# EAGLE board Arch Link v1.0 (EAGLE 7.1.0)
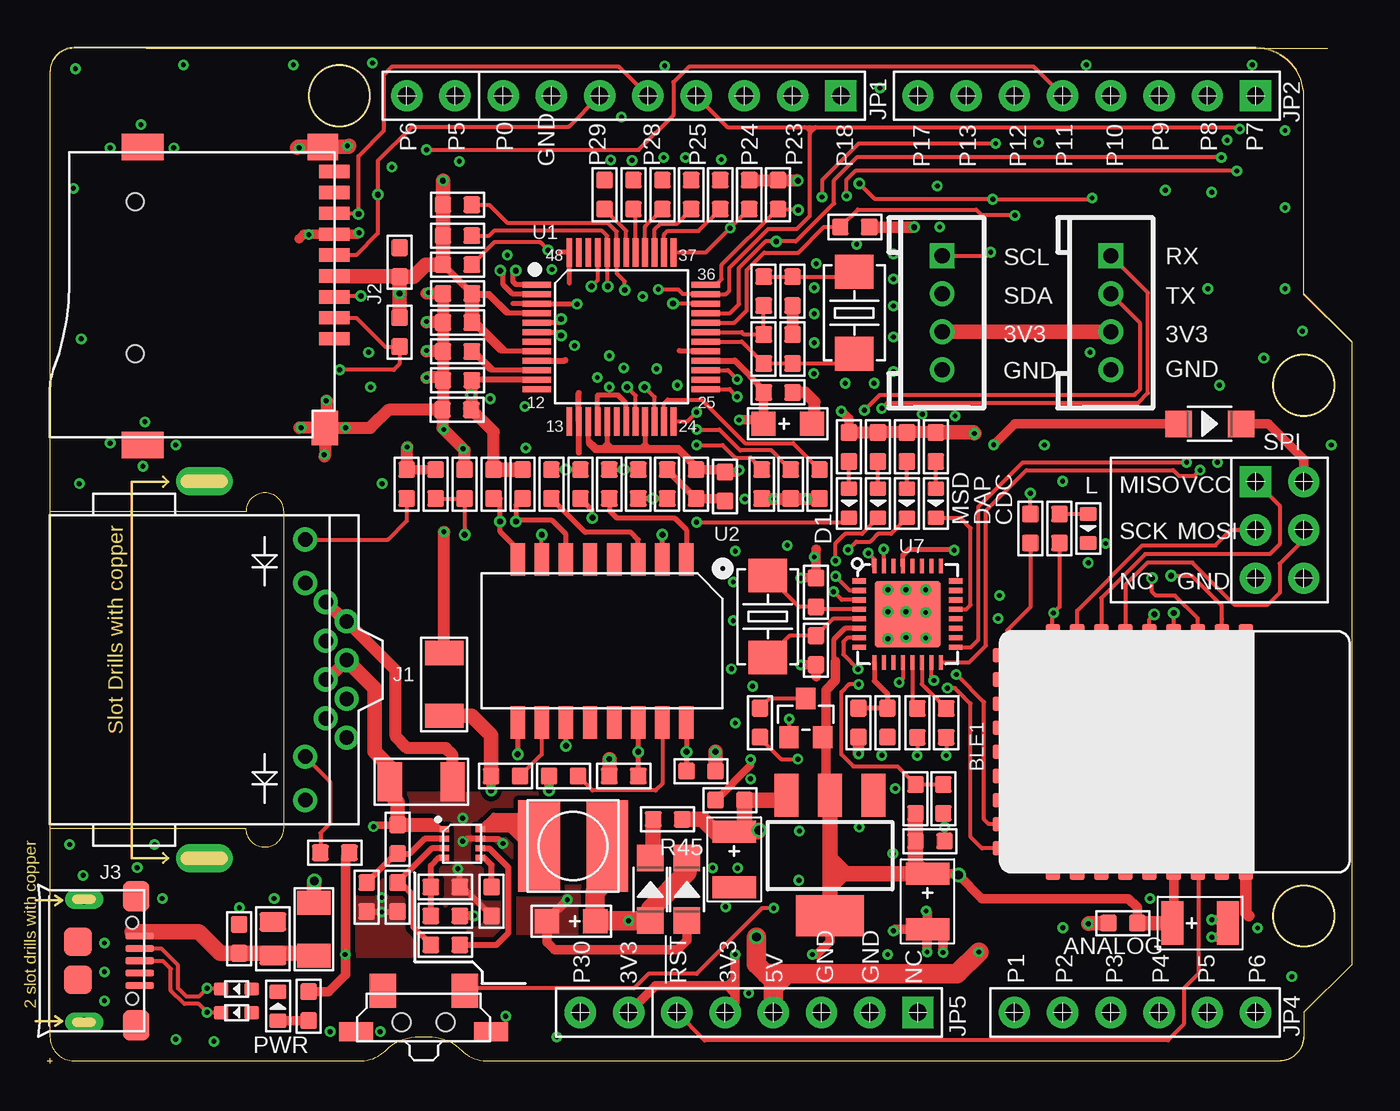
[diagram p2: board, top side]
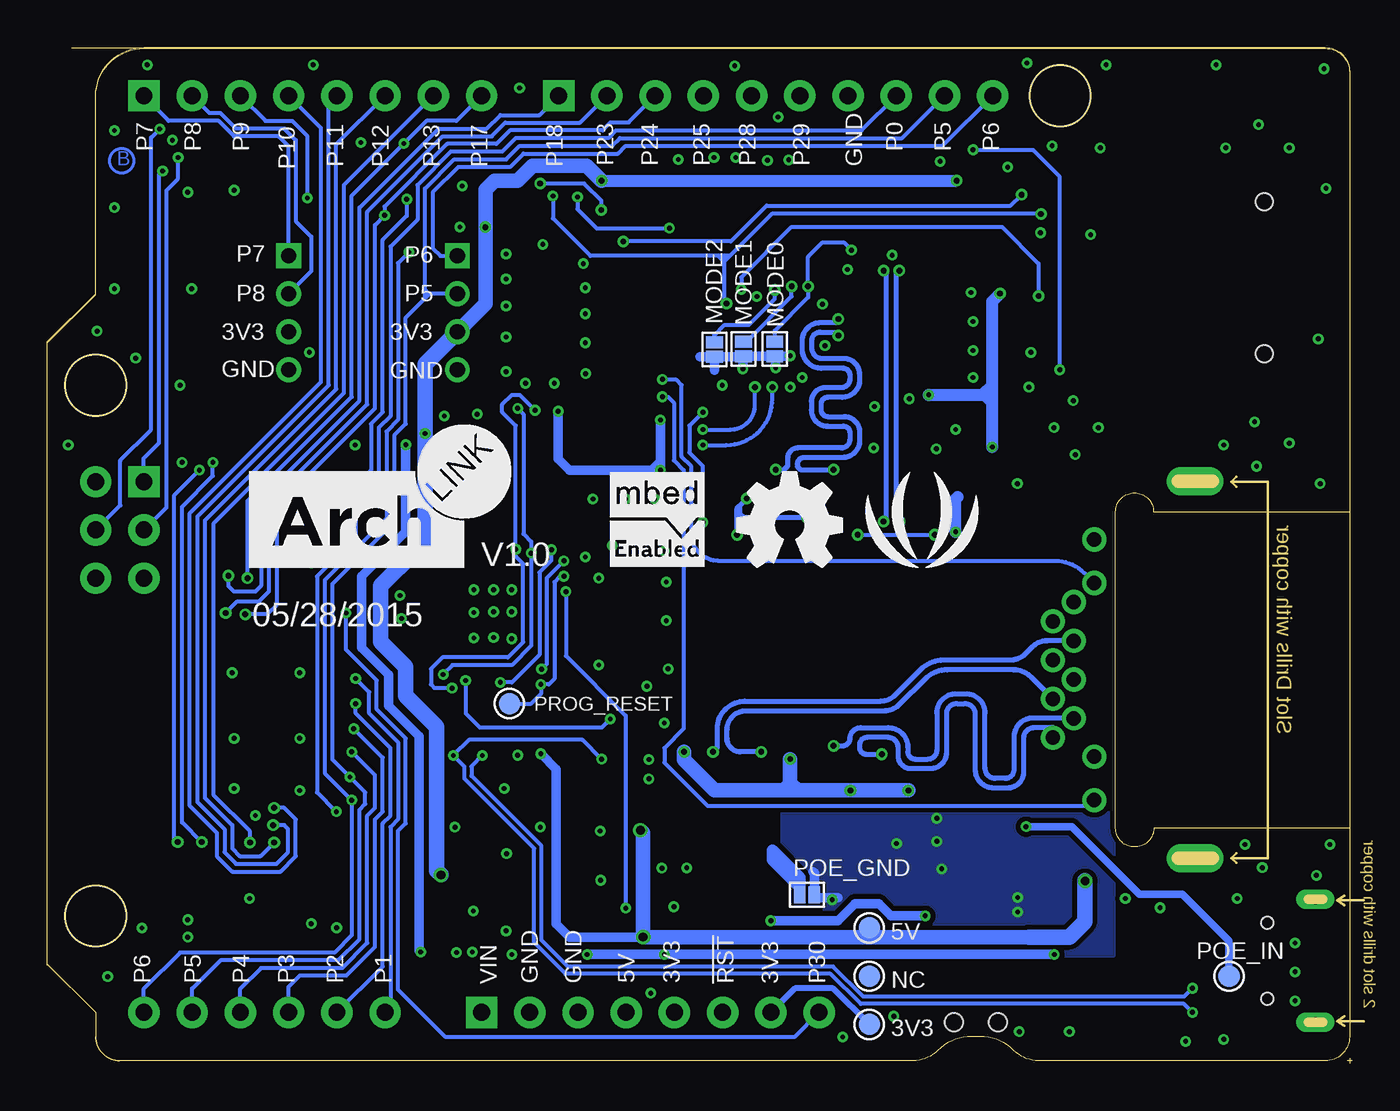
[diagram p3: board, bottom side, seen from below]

Size 68.71 x 53.47 mm. Coordinates in mm from the lower left corner, seen from the top.
Outline: 1.4,53.42 arc90 0.13,52.15
Outline: 66.17,50.88 arc90 63.63,53.42
Outline: 1.4,53.42 arc90 0.13,52.15
Outline: 66.17,50.88 arc90 63.63,53.42
Outline: 1.4,53.42 arc90 0.13,52.15
Outline: 66.17,50.88 arc90 63.63,53.42
Outline: 5.21,53.42 67.44,53.42
Outline: 1.4,53.42 arc90 0.13,52.15
Outline: 66.17,50.88 arc90 63.63,53.42
Outline: 63.63,53.42 1.4,53.42
Outline: 1.4,53.42 arc90 0.13,52.15
Outline: 68.71,5.16 68.71,37.92 66.17,40.46 66.17,50.88
Outline: 66.17,50.88 arc90 63.63,53.42
Outline: circle at 15.37,50.93 radius 1.61
Outline: circle at 66.17,7.75 radius 1.61
Outline: circle at 66.17,35.69 radius 1.61
Copper layers (1*16): Top 0.035mm / dielectric 1.5mm / Bottom 0.035mm
Design rules "SeeedStudio_2layer_DRU_no_angle_20140221 *": minimum track width 6mil, minimum drill 10mil, track to track 6mil, track to pad 6mil, pad to pad 6mil, via to via 6mil, smd to smd 0mil, copper to edge 10mil, drill to drill 10mil, minimum pad ring 10mil, minimum via ring 6mil, stop-mask expansion 2mil, vias tented up to drill 25mil, thermal gap 10mil
tRestrict: area 26.9,9.7 to 28.3,13.2; area 62.4,9 to 68.7,23.6
bRestrict: area 62.4,9 to 68.7,23.6

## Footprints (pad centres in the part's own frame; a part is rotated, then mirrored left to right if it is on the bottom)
TP-D45MIL = smd 1.143 x 1.143: T 0,0
SEEED_BLE_MODULE_PAD = smd 1.524 x 0.762: 1 -5.969,12.954; 2 -5.969,11.684; 3 -5.969,10.414; 4 -5.969,9.144; 5 -5.969,7.874; 6 -5.969,6.604; 7 -5.969,5.334; 8 -5.969,4.064; 9 -5.969,2.794; 19 5.969,2.794; 20 5.969,4.064; 21 5.969,5.334; 22 5.969,6.604; 23 5.969,7.874; 24 5.969,9.144; 25 5.969,10.414; 26 5.969,11.684; 27 5.969,12.954 | smd 0.762 x 1.524: 10 -5.08,0.381; 11 -3.81,0.381; 12 -2.54,0.381; 13 -1.27,0.381; 14 0,0.381; 15 1.27,0.381; 16 2.54,0.381; 17 3.81,0.381; 18 5.08,0.381
C0603 = smd 0.889 x 0.889: 1 0,0.762; 2 0,-0.762
AVX-A = smd 1.27 x 1.27: + -1.27,0; - 1.27,0
C1206 = smd 1.27 x 2.032: 1 -1.651,0; 2 1.651,0
AVX-B = smd 1.143 x 2.286: + -1.46,0; - 1.46,0
C0805 = smd 1.397 x 1.016: 1 0,0.889; 2 0,-0.889
LED-0603 = smd 0.762 x 0.889: + -0.762,0; - 0.762,0
SOD-123 = smd 1.397 x 1.397: + -1.651,0; - 1.651,0
SOD-523 = smd 0.762 x 0.7: + -0.8,0; - 0.8,0
F1206 = smd 1.27 x 1.778: 1 -1.397,0; 2 1.397,0
HW4-2.0 = drill 0.8 pad 1.27 square: 1 -3,0 | drill 0.8 pad 1.27: 2 -1,0; 3 1,0; 4 3,0
RJ45-12+2P-16.3X15.4X11.5MM-IN = drill 0.762 pad 1.27: 1 3.57,7.5; 2 2.55,6.4; 3 1.53,7.5; 4 0.51,6.4; 5 -0.51,7.5; 6 -1.53,6.4; 7 -2.55,7.5; 8 -3.57,6.4; 9 6.86,5.32; 10 4.57,5.32; 11 -4.57,5.32; 12 -6.86,5.32 | drill 0.6 pad 1.5 long: 13 -9.92,0; 14 9.92,0
MICRO-SD9+4P-SMD-16.1X14.5X1.85MM = smd 1.6 x 0.7: 1 0,2.25; 2 0,1.15; 3 0,0.05; 4 0,-1.05; 5 0,-2.15; 6 0,-3.25; 7 0,-4.35; 8 0,-5.45; 9 0,-6.55 | smd 1.6 x 1.4: G1 0.6,-7.85 | smd 2.2 x 1.4: G2 10.1,-7.85; G3 10.1,7.85 | smd 1.4 x 1.8: G4 0.5,6.95 | hole 0.9: 10.5,-4.95; 10.5,3.05
MICRO-USB5+4P-SMD-0.65-B = smd 0.381 x 1.524: 1 -1.3,-0.25; 2 -0.65,-0.25; 3 0,-0.25; 4 0.65,-0.25; 5 1.3,-0.25 | smd 1.6 x 1.397: S1 -3.4,-0.427; S6 3.4,-0.427 | drill 0.508 pad 1.016 long: S2 -3.226,-3.175; S5 3.226,-3.175 | smd 1.5 x 1.5: S3 -1,-3.5; S4 1,-3.5 | hole 0.635: -2,-0.65; 2,-0.65
INT2-SMD-4.8X4.8X3MM = smd 2.2 x 4.8: 1 -1.8,0; 2 1.8,0
JUMPER-2P = smd 0.889 x 0.61: 1 0,0.381; 2 0,-0.381
SOT-23 = smd 1.016 x 1.143: 1 -0.889,-1.016; 2 0.889,-1.016; 3 0,1.016
R0603 = smd 0.889 x 0.889: 1 0,0.762; 2 0,-0.762
SW4-SMD-7.0X3.5X3.5MM-90D = smd 1.397 x 1.778: 1 -2.159,1.651; 2 2.159,1.651 | smd 1.778 x 1.016: S1 -3.556,-0.508; S2 3.556,-0.508 | hole 0.95: -1.15,0; 1.15,0
LQFP48-0.5-7X7MM = smd 1.5 x 0.3: 1 -4.45,2.75; 2 -4.45,2.25; 3 -4.45,1.75; 4 -4.45,1.25; 5 -4.45,0.75; 6 -4.45,0.25; 7 -4.45,-0.25; 8 -4.45,-0.75; 9 -4.45,-1.25; 10 -4.45,-1.75; 11 -4.45,-2.25; 12 -4.45,-2.75; 25 4.45,-2.75; 26 4.45,-2.25; 27 4.45,-1.75; 28 4.45,-1.25; 29 4.45,-0.75; 30 4.45,-0.25; 31 4.45,0.25; 32 4.45,0.75; 33 4.45,1.25; 34 4.45,1.75; 35 4.45,2.25; 36 4.45,2.75 | smd 0.3 x 1.5: 13 -2.75,-4.45; 14 -2.25,-4.45; 15 -1.75,-4.45; 16 -1.25,-4.45; 17 -0.75,-4.45; 18 -0.25,-4.45; 19 0.25,-4.45; 20 0.75,-4.45; 21 1.25,-4.45; 22 1.75,-4.45; 23 2.25,-4.45; 24 2.75,-4.45; 37 2.75,4.45; 38 2.25,4.45; 39 1.75,4.45; 40 1.25,4.45; 41 0.75,4.45; 42 0.25,4.45; 43 -0.25,4.45; 44 -0.75,4.45; 45 -1.25,4.45; 46 -1.75,4.45; 47 -2.25,4.45; 48 -2.75,4.45
SOIC16-1.27-12.7X7.0MM = smd 0.762 x 1.714: 1 -4.445,-4.286; 2 -3.175,-4.286; 3 -1.905,-4.286; 4 -0.635,-4.286; 5 0.635,-4.286; 6 1.905,-4.286; 7 3.175,-4.286; 8 4.445,-4.286; 9 4.445,4.286; 10 3.175,4.286; 11 1.905,4.286; 12 0.635,4.286; 13 -0.635,4.286; 14 -1.905,4.286; 15 -3.175,4.286; 16 -4.445,4.286
SEEEDUINO-ARDUINO-DIM = drill 0.889 pad 1.651 square: 1 63.5,50.8; 9 41.656,50.8; 25 45.72,2.54; 44 63.5,30.48 | drill 0.889 pad 1.651: 2 60.96,50.8; 3 58.42,50.8; 4 55.88,50.8; 5 53.34,50.8; 6 50.8,50.8; 7 48.26,50.8; 8 45.72,50.8; 10 39.116,50.8; 11 36.576,50.8; 12 34.036,50.8; 13 31.496,50.8; 14 28.956,50.8; 15 26.416,50.8; 16 23.876,50.8; 17 21.336,50.8; 18 18.796,50.8; 19 50.8,2.54; 20 53.34,2.54; 21 55.88,2.54; 22 58.42,2.54; 23 60.96,2.54; 24 63.5,2.54; 26 43.18,2.54; 27 40.64,2.54; 28 38.1,2.54; 29 35.56,2.54; 30 33.02,2.54; 31 30.48,2.54; 32 27.94,2.54; 39 66.04,30.48; 40 63.5,27.94; 41 63.5,25.4; 42 66.04,25.4; 43 66.04,27.94 | hole 3.2: 15.24,50.8; 66.04,35.56; 66.04,7.62
SOT-223 = smd 1.27 x 2.286: 1 -2.286,-3.175; 2 0,-3.175; 3 2.286,-3.175 | smd 3.556 x 2.159: TER 0,3.175
TDFN8-0.5-2X2MM = smd 0.5 x 0.3: 1 -0.95,0.75; 2 -0.95,0.25; 3 -0.95,-0.25; 4 -0.95,-0.75; 5 0.95,-0.75; 6 0.95,-0.25; 7 0.95,0.25; 8 0.95,0.75
HVQFN33 = smd 0.762 x 0.279: 1 -2.54,1.75; 2 -2.54,1.25; 3 -2.54,0.75; 4 -2.54,0.25; 5 -2.54,-0.25; 6 -2.54,-0.75; 7 -2.54,-1.25; 8 -2.54,-1.75; 17 2.54,-1.75; 18 2.54,-1.25; 19 2.54,-0.75; 20 2.54,-0.25; 21 2.54,0.25; 22 2.54,0.75; 23 2.54,1.25; 24 2.54,1.75 | smd 0.279 x 0.762: 9 -1.75,-2.54; 10 -1.25,-2.54; 11 -0.75,-2.54; 12 -0.25,-2.54; 13 0.25,-2.54; 14 0.75,-2.54; 15 1.25,-2.54; 16 1.75,-2.54; 25 1.75,2.54; 26 1.25,2.54; 27 0.75,2.54; 28 0.25,2.54; 29 -0.25,2.54; 30 -0.75,2.54; 31 -1.25,2.54; 32 -1.75,2.54 | smd 3.5 x 3.5: 33 0,0
X2-SMD-5.0X3.2X1.3MM = smd 1.778 x 2.032: 1 -2.159,0; 2 2.159,0

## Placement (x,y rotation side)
3V3  [TP-D45MIL]  25.43,2.03 0 bottom
5V  [TP-D45MIL]  25.43,7.11 0 bottom
BLE1  BLE Nano  [SEEED_BLE_MODULE_PAD]  50.16,16.38 270 top
C1  100nF  [C0603]  21.59,35.94 90 top
C2  100nF  [C0603]  21.59,38.99 90 top
C3  100nF  [C0603]  21.59,40.51 90 top
C4  100nF  [C0603]  34.16,30.48 180 top
C5  100nF  [C0603]  21.56,34.39 90 top
C6  100nF  [C0603]  35.69,30.35 180 top
C7  4.7uF  [C0603]  37.62,30.48 180 top
C8  10nF  [C0603]  39.14,30.48 180 top
C9  10uF/16V  [AVX-A]  38.99,33.66 0 top
C10  100nF  [C0603]  38.48,35.31 270 top
C11  22pF  [C0603]  39.24,37.59 0 top
C12  22pF  [C0603]  39.24,40.64 180 top
C13  1nF/1000V  [C1206]  20.89,19.94 270 top
C14  6.8nF  [C0603]  26.54,30.48 0 top
C15  6.8nF  [C0603]  29.59,30.48 0 top
C16  10nF  [C0603]  32.64,30.48 0 top
C17  22nF  [C0603]  21.97,30.48 180 top
C18  100nF  [C0603]  35.94,13.84 90 top
C19  22uF/10V  [AVX-B]  36.17,10.72 270 top
C20  22uF/10V  [AVX-B]  46.35,8.51 270 top
C21  100nF  [C0603]  46.48,11.68 270 top
C22  100nF  [C0603]  18.54,42.16 0 top
C23  NC/1uF  [C0603]  18.44,8.74 180 top
C24  22uF/10V  [AVX-B]  60.71,7.37 0 top
C25  100nF  [C0603]  10.1,6.54 0 top
C26  10uF  [C0805]  11.87,6.54 0 top
C27  18pF  [C0603]  40.47,24.78 0 top
C28  18pF  [C0603]  40.47,21.73 180 top
C29  100nF  [C0603]  47.18,13.91 180 top
C30  100nF  [C0603]  56.64,7.37 90 top
C31  NC/10uF/25V  [AVX-A]  27.58,7.47 180 top
C32  NC/1uF/100v  [C1206]  19.68,14.81 180 top
CDC  RED  [LED-0603]  46.79,29.46 270 top
D1  RED  [LED-0603]  42.21,29.46 270 top
D2  B0540W  [SOD-123]  31.75,9.14 90 top
D4  CG0603MLC-05E  [SOD-523]  9.96,2.65 180 top
D5  B0540W  [SOD-123]  61.21,33.66 0 top
D6  CG0603MLC-05E  [SOD-523]  9.96,3.9 180 top
D7  NC/304060001  [SOD-123]  33.68,9.14 90 top
DAP  BLUE  [LED-0603]  45.26,29.46 270 top
F1  PPTC_750mA  [F1206]  14.03,7.05 90 top
I2C  320110033  [HW4-2.0]  47.12,39.5 270 top
J1  MJ88-BX11-RVSL2  [RJ45-12+2P-16.3X15.4X11.5MM-IN]  8.26,20.7 270 top
J2  320090008  [MICRO-SD9+4P-SMD-16.1X14.5X1.85MM]  15.11,40.39 180 top
J3  ST-USB-001G  [MICRO-USB5+4P-SMD-0.65-B]  5.11,5.38 270 top
L  BLUE  [LED-0603]  54.81,28.14 270 top
L1  NC/33uH  [INT2-SMD-4.8X4.8X3MM]  27.69,11.43 0 top
MODE0  NC  [JUMPER-2P]  30.4,37.59 0 bottom
MODE1  NC  [JUMPER-2P]  32.05,37.59 0 bottom
MODE2  NC  [JUMPER-2P]  33.58,37.57 0 bottom
MSD  YELLOW  [LED-0603]  43.74,29.46 270 top
NC  [TP-D45MIL]  25.43,4.57 0 bottom
POE_GND  NC  [JUMPER-2P]  28.7,8.86 270 bottom
POE_IN  DNP  [TP-D45MIL]  6.48,4.57 0 bottom
PROG_RESET  NC  [TP-D45MIL]  44.37,18.92 0 bottom
PWR  GREEN  [LED-0603]  12.14,3 90 top
Q1  CJ2305  [SOT-23]  39.94,18.17 0 top
R1  12.4k/1%  [R0603]  21.59,37.47 90 top
R2  47k  [R0603]  40.67,30.48 180 top
R3  1M  [R0603]  37.72,37.59 0 top
R4  0R  [R0603]  37.72,40.64 180 top
R5  10K  [R0603]  42.52,44.02 270 top
R6  10K  [R0603]  38.48,45.72 0 top
R7  10K  [R0603]  36.96,45.72 0 top
R8  47K  [R0603]  35.43,45.72 0 top
R9  47K  [R0603]  33.91,45.72 0 top
R10  47K  [R0603]  32.38,45.72 0 top
R11  47K  [R0603]  30.86,45.72 0 top
R12  47K  [R0603]  29.34,45.72 0 top
R13  47K  [R0603]  21.59,42.04 90 top
R14  47K  [R0603]  21.59,43.56 90 top
R15  47K  [R0603]  21.59,45.19 90 top
R16  1K  [R0603]  18.92,30.48 180 top
R17  1K  [R0603]  15.14,11.07 90 top
R18  1K  [R0603]  42.21,32.44 180 top
R19  75R/1%  [R0603]  24.13,15.11 270 top
R20  75R/1%  [R0603]  27.18,15.11 270 top
R21  150R/1%  [R0603]  30.35,15.11 270 top
R22  150R/1%  [R0603]  34.42,15.37 270 top
R23  49.9R/1%  [R0603]  23.5,30.48 0 top
R24  49.9R/1%  [R0603]  25.02,30.48 0 top
R25  10R/1%  [R0603]  20.45,30.48 0 top
R26  82R/1%  [R0603]  31.11,30.48 0 top
R27  82R/1%  [R0603]  28.07,30.48 0 top
R28  1k  [R0603]  13.75,3 180 top
R29  10K  [R0603]  18.54,38.48 0 top
R30  NC/1M  [R0603]  18.44,11.79 180 top
R31  NC/110K  [R0603]  16.81,8.74 180 top
R32  NC/1K  [R0603]  20.96,6.22 90 top
R33  NC/510K/1%  [R0603]  20.96,7.75 270 top
R34  NC/100K/1%  [R0603]  20.96,9.27 90 top
R35  NC/0R  [R0603]  23.39,8.51 0 top
R36  33R  [R0603]  47.33,17.91 180 top
R37  33R  [R0603]  45.81,17.91 180 top
R38  1.5K  [R0603]  37.53,17.92 180 top
R39  10K  [R0603]  45.72,13.91 0 top
R40  10K  [R0603]  42.71,17.92 180 top
R41  15K  [R0603]  44.23,17.92 180 top
R42  1K  [R0603]  46.79,32.44 180 top
R43  1K  [R0603]  43.74,32.44 180 top
R44  1K  [R0603]  45.26,32.44 180 top
R45  NC/0R  [R0603]  32.66,12.83 90 top
R46  0R  [R0603]  51.77,28.14 180 top
R47  3.3K  [R0603]  53.3,28.14 0 top
RESET  311020023  [SW4-SMD-7.0X3.5X3.5MM-90D]  19.81,2.16 0 top
U1  W5500  [LQFP48-0.5-7X7MM]  30.23,38.23 0 top
U2  HST-0041S  [SOIC16-1.27-12.7X7.0MM]  29.21,22.22 180 top
U3  DNP  [SEEEDUINO-ARDUINO-DIM]  0.13,0.13 0 top
U4  CJ1117-3.3  [SOT-223]  41.21,10.92 180 top
U5  NC/MAX1502C  [TDFN8-0.5-2X2MM]  21.84,11.56 0 top
U7  LPC11U35FHI33-5X5  [HVQFN33]  45.3,23.63 0 top
U$1  [SEEEDSTUDIO-PCB-FRAME]  not placed on the board
U$20  [SEEEDSTUDIO-PCB-FRAME]  not placed on the board
U$34  [SEEEDSTUDIO-PCB-FRAME]  not placed on the board
U$38  [SEEEDSTUDIO-PCB-FRAME]  not placed on the board
UART  320110033  [HW4-2.0]  56.01,39.5 270 top
X1  25MHz/306010064  [X2-SMD-5.0X3.2X1.3MM]  42.49,39.5 90 top
X2  12MHz/306010047  [X2-SMD-5.0X3.2X1.3MM]  37.93,23.51 90 top

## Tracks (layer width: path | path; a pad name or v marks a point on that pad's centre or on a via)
1
  Top 0.203: U1.23 32.48,34.74 32.66,34.93 34.44,34.93 36.73,32.64 39.27,32.64 R2.2
1V2O  (via drill 0.25 pad 0.51, 0.3 pad 0.51)
  Top 0.203: U1.22 31.98,35.05 v31.45,35.59 | C8.2 38.13,32.26 36.47,32.26 35.38,33.35 v34.19,33.35
  Bottom 0.203: v34.19,33.35 32.74,33.35 arc-90 31.45,34.64 v31.45,35.59
2
  Top 0.203: U1.38 32.48,43.63 32.66,43.82 34.29,43.82 R8.2
3
  Top 0.203: U1.39 31.98,43.89 32.28,44.2 33.15,44.2 R9.2 33.78,44.96
3V3  (via drill 0.25 pad 0.41, 0.25 pad 0.51, 0.3 pad 0.51, 0.46 pad 0.76)
  Top 0.203: 29.62,32.23 28.82,32.23 28.48,32.58 U1.15 28.48,32.87 28.91,32.44 29.31,32.44 29.72,32.44 | 29.62,32.23 31.55,32.23 | 31.55,32.23 33.17,32.23 C4.2 | 29.62,32.23 29.48,32.37 29.48,32.64 29.52,32.64 29.72,32.44 | 31.48,32.3 31.55,32.23 | 29.72,32.44 31.45,32.44 33.24,32.44 34.29,31.39 34.29,31.11 | 22.33,35.92 C1.2 | C2.2 22.35,39.19 | R42.2 46.05,33.2 46.02,33.22 | U1.11 22.42,35.98 22.4,35.99 22.4,35.28 v22.3,35.18 22.5,34.98 | C9.+ 37.72,33.76 37.62,33.86
  Top 0.254: U7.29 45.05,26.74 45.36,27.05 47.7,27.05 v47.75,27 | U1.15 28.48,32.66 28.8,32.33 | U1.17 29.48,32.64 29.48,32.6 29.31,32.44 | U1.21 31.48,32.61 | 31.48,32.57 31.48,32.47 31.45,32.44 | 31.48,32.61 31.48,32.57 | 31.48,32.57 31.24,32.33 | 31.48,32.61 31.75,32.33 | 24.02,37.48 23.86,37.48 C2.2 | 24.3,39.48 23.27,40.51 C3.2 | U1.4 24.3,39.48 | 24.3,39.48 24.18,39.48 23.27,40.39 22.5,40.39 | 24.14,37.48 24.02,37.48 | 24.02,37.48 22.63,38.86 22.63,38.99 | U1.8 24.14,37.48 | 24.14,37.48 22.63,38.99 | 22.63,38.99 22.5,39.12 | U7.6 42.01,22.88 41.4,22.28 41.4,21.26 41.5,21.16
  Top 0.305: U1.28 36.2,36.98 37.72,35.46 C10.2 | U1.11 22.39,35.98 C1.2
  Top 0.381: C3.2 R13.1
  Top 0.508: R25.1 R16.2 | BLE1.24 59.31,7.3 | C30.2 57.4,8.19 56.94,8.66 49.23,8.66 v47.98,9.91 47.92,9.97 C20.+ | C10.2 C9.+ | 36.4,31.24 v36.42,31.22 36.32,31.11 C6.2 35.56,31.24 C4.2 | v36.42,33.86 37.62,33.86 37.67,33.86 | 40.79,17.12 Q1.2 41,17.32 | 41.5,21.16 41.5,20.14 41,19.63 41,17.32 | R18.2 42.21,33.91 v41.81,34.32 | 59.31,6.92 59.31,7.3 | 59.31,7.3 C24.+ | 15.7,5.7 15.7,10.87 R17.2 | U4.2 41.21,14.22 | 41.21,14.22 41.21,14.57 | U4.TER 41.21,6.39 40.54,5.71 v40.28,5.71 | R28.2 14.81,3.76 15.7,4.64 15.7,5.7 | 15.7,5.7 v15.68,5.71 | 41,17.32 41,14.44 41.21,14.22 | v36.22,5.71 36.22,4.44 | 36.22,4.44 36.22,4.19 | 36.22,3.68 36.22,3.2 U3.29 | U3.31 30.63,2.67 32.03,4.06 35.84,4.06 | 35.84,4.06 36.09,4.06 36.22,4.19 | 35.84,4.06 36.22,4.44 | 35.84,4.06 36.22,3.68 | 36.22,3.68 36.22,4.19
  Top 0.61: v45.64,44.01 43.29,44.01 R5.1
  Top 0.635: 22.2,34.47 22.25,34.52 22.25,34.47 C5.2 | R16.2 18.95,31.27 v18.95,32.44 | 22.33,35.92 22.33,35.2 v22.3,35.18 22.33,35.15 C5.2 | R23.1 23.5,33.22 C5.2 | R18.2 R43.2 R44.2 R42.2 | R7.1 R6.1 39.5,46.48 v39.52,46.46
  Top 0.762: UART.3 I2C.3 | J2.4 18.54,41.44 C22.2 | v20.83,46.46 R15.1 R14.1 R13.1 19.91,42.04 19.28,41.4 C22.2 | C22.2 v18.54,40.51 R29.1 | C3.2 22.35,39.19 22.4,39.14 | R24.1 R23.1 | C30.2 C24.+ | R42.2 48.77,33.2 v48.82,33.15
  Top 0.813: U4.TER 41.21,10.03 | 41.21,10.03 41.21,14.22 | C20.+ 46.25,9.97 | 46.25,9.97 42,9.97 | 41.87,9.97 41.28,9.97 41.21,10.03 | 46.25,9.97 45.72,10.5 C21.2 R39.2 | 42,9.97 41.3,10.67 | 42,9.97 41.87,9.97 | 41.87,9.97 41.3,9.4
  Bottom 0.305: 3V3.T 27.33,3.94 29.34,3.94 U3.31
  Bottom 0.508: v40.28,5.71 v36.22,5.71 v15.68,5.71 | v36.42,31.22 36.42,31.67 | 36.42,31.67 v36.42,33.86 | v36.42,31.22 36.45,31.24 36.86,31.24 36.42,31.67 | v41.81,34.32 41.81,31.83 41.2,31.22 v36.42,31.22 | v47.75,27 48.26,27 | 48.26,27 49.28,27 49.33,26.95 | 48.26,27 48.82,27.56
  Bottom 0.635: v18.95,32.44 18.95,34.77 | 18.95,34.77 18.95,35.69 | 18.95,35.69 18.95,40.11 v18.54,40.51 | v22.3,35.18 19.46,35.18 | 19.46,35.18 19.35,35.18 18.95,34.77 | 19.46,35.18 18.95,35.69 | v39.52,46.46 v20.83,46.46
  Bottom 0.762: I2C.3 45.64,39.97 v45.64,44.01 45.64,45.97 45.16,46.46 43.94,46.46 43.15,47.24 40.31,47.24 v39.52,46.46
  Bottom 0.813: I2C.3 48.82,36.8 v48.82,33.15 48.82,27.56 48.82,27.46 49.33,26.95 51.16,25.12 51.16,22.17 49.83,20.85 49.83,19.33 48.21,17.7 48.21,10.13 v47.98,9.91
4
  Top 0.203: U1.40 31.48,44.05 R10.2
5
  Top 0.203: U1.41 30.98,44.84 R11.2
5V  (via drill 0.25 pad 0.51, 0.46 pad 0.76)
  Top 0.508: D5.+ 50.94,33.66 v49.83,32.55
  Top 0.61: v42.72,16.28 42.72,17.14 R40.1
  Top 0.762: F1.2 14.03,9.56 v14.06,9.59
  Top 0.813: U4.3 38.67,13.84 C18.2 36.7,12.21 36.73,12.18 | C19.+ 36.35,12.18 | 36.35,12.18 36.73,12.18 | 36.73,12.18 37.4,12.18 v37.48,12.26 | R45.2 34.51,12.83 35.27,12.07 36.23,12.07 36.35,12.18
  Top 1.016: 37.85,4.7 47.9,4.7 v49.05,5.84 | 37.85,4.7 37.34,5.21 v37.34,6.63 | U3.28 38.23,3.99 | 38.23,3.99 38.23,4.32 37.85,4.7 | 38.23,3.99 38.25,3.99 38.86,4.6
  Bottom 0.203: 17.02,6.63 24.94,6.63 5V.T
  Bottom 0.508: v37.34,6.63 41.2,6.63 41.91,7.34 41.91,15.47 v42.72,16.28 | v49.83,32.55 49.83,27.96 52.17,25.63 52.17,21.87 50.75,20.45 50.75,18.82 49.12,17.2 49.12,5.92 v49.05,5.84
  Bottom 0.762: 17.02,6.63 v37.34,6.63 37.34,12.12 v37.48,12.26
  Bottom 0.813: 17.02,6.63 14.88,6.63 14.07,7.44 v14.07,9.58 v14.06,9.59
6
  Top 0.203: U1.42 30.48,43.82 R12.2
ACTLED  (via drill 0.25 pad 0.51)
  Top 0.203: U1.27 35.84,36.48 v36.32,35.99
  Bottom 0.203: v36.32,35.99 35.61,35.99 35.31,35.69 35.31,31.93 34.8,31.42 34.8,27.87 arc-90 33.37,26.44 15.65,26.44 arc45 14.11,25.8 J1.11
AGND  (via drill 0.25 pad 0.51)
  Top 0.203: C23.1 18.16,7.98 18.14,7.95
  Top 0.305: R35.2 21.87,9.27 R34.2 21.72,10.12 v21.62,10.22 | 22.12,11.81 U5.7 23.74,11.81 v23.99,11.56 | R31.1 C23.1 | 18.14,7.95 v17.61,7.95
  Top 0.508: v27.38,8.6 26.31,7.53 C31.- 26.31,6.35 26.7,5.97 33.17,5.97 33.68,6.48 D7.+
  Top 0.635: C32.1 21.34,16.23 20.98,16.59 18.95,16.59 18.34,17.2 18.34,20.67 J1.7 15.68,23.25 J1.8
  Bottom 0.508: 27.08,8.7 28.16,8.7 POE_GND.1 28.32,10.01 28.4,10.08
  other vias: 21.87,12.89 21.87,11.67 17.61,8.71
  pour Top (isolate 0.254, no thermals): 12.55,14.2 12.55,5.61 23.93,5.61 24.23,5.92 24.23,6.83 30.02,6.83 30.02,14.2
  pour Bottom (isolate 0.254, no thermals): 12.55,14.34 12.55,5.61 23.93,5.61 24.23,5.92 24.23,6.83 30.02,6.83 30.02,14.14
BLE_MISO  (via drill 0.25 pad 0.51, 0.3 pad 0.51)
  Top 0.203: J2.7 16.35,44.74 v16.38,44.7 16.38,47.75 17.73,49.1 17.73,52.05 18.14,52.45 30.1,52.45 U3.13 | BLE1.7 55.5,24.48 57.82,26.8 64.39,26.8 64.9,27.3 64.9,29.34 U3.44 | U1.34 32.96,39.98 v32.94,39.99 | v62.64,46.97 42.55,46.97 42.06,46.48 42.06,45.67 v42.09,45.64
  Bottom 0.203: v16.38,44.7 30.56,44.7 32.77,42.49 | 32.77,42.49 33.17,42.49 | 33.17,42.49 40.11,42.49 42.09,44.48 v42.09,45.64 | 33.07,42.19 32.77,42.49 | 33.07,42.19 33.07,42.39 33.17,42.49 | U3.44 63.65,30.63 63.65,31.83 62.84,32.64 62.84,46.76 v62.64,46.97 | 33.07,42.19 33.07,40.12 v32.94,39.99 | 33.07,42.19 33.36,42.48
BLE_MOSI  (via drill 0.25 pad 0.51, 0.3 pad 0.51)
  Top 0.152: 39.88,49.28 40.18,48.98 40.18,48.9
  Top 0.203: J2.3 15.16,40.39 v16.51,40.39 | U3.12 35.81,49.28 39.88,49.28 40.16,49.28 | U3.43 66.17,27.56 64.9,26.29 64.9,24.77 64.26,24.13 62.51,24.13 60.3,26.34 57.93,26.34 56.77,25.17 BLE1.6 | 40.16,49.28 40.46,49.28 | 40.46,49.28 62.69,49.28 v62.79,49.17 | 40.16,48.97 40.16,44.6 39.47,43.92 37.97,43.92 35.92,41.86 35.92,40.66 35.73,40.48 U1.35 33.46,40.48 33.21,40.73 v32.17,40.73 | 40.16,48.97 40.16,49.28 | 40.46,49.28 40.16,48.97
  Bottom 0.203: U3.43 64.87,29.36 64.87,31.72 63.25,33.35 63.25,48.72 v62.79,49.17 | v16.51,40.39 16.51,42.09 18.44,44.02 29.51,44.02 32.17,41.37 v32.17,40.73
BLE_RX  (via drill 0.25 pad 0.41, 0.25 pad 0.51)
  Top 0.203: BLE1.17 49.58,12.57 49.33,12.83 49.33,19 v47.87,20.46 | v43.94,34.47 44.25,34.77 57.45,34.77 57.96,35.28 57.96,40.54 UART.1 | U7.32 43.51,26.14 43.51,26.57 v43.23,26.85
  Bottom 0.203: U3.1 63.63,50.9 62.33,49.61 59.69,49.61 58.88,48.79 56.54,48.79 56.01,48.26 UART.1 | v47.87,20.46 47.37,20.95 44.25,20.95 43.23,21.97 v43.23,26.85 43.23,27.46 43.64,27.86 43.64,34.16 v43.94,34.47
BLE_SCL  (via drill 0.25 pad 0.51)
  Top 0.203: v52.68,13.84 BLE1.16 | I2C.1 49.48,42.5 v49.67,42.69
  Bottom 0.203: U3.24 63.63,3.91 61.72,5.82 53.59,5.82 52.68,6.73 v52.68,13.84 54.1,15.27 54.1,25.42 50.85,28.68 50.85,33.25 50.24,33.86 50.24,42.11 v49.67,42.69 | I2C.1 48.01,42.49 48.41,42.9 48.41,45.84 47.08,47.17 44.35,47.17 43.64,47.88 38.66,47.88 38.25,48.29 21.56,48.29 U3.18
BLE_SCLK  (via drill 0.25 pad 0.51, 0.3 pad 0.51)
  Top 0.203: J2.5 16.26,42.54 17.4,43.68 v17.4,45.72 17.4,47.5 19.2,49.3 27.46,49.3 U3.14 | BLE1.8 54.23,23.82 57.66,27.25 61.52,27.25 62.33,28.07 U3.40 | U1.33 35.95,39.48 36.42,39.95 36.42,41.86 37.82,43.26 v38.38,43.26 39.42,43.26 41.43,45.26 41.43,46.48 42.62,47.68 v61.82,47.68
  Bottom 0.203: v38.38,43.26 32.72,43.26 30.84,45.14 17.98,45.14 v17.4,45.72 | U3.40 62.43,29.26 62.43,45.95 61.82,46.56 v61.82,47.68
BLE_SDA  (via drill 0.25 pad 0.51)
  Top 0.203: v52.78,15.06 50.6,15.06 BLE1.15 50.5,15.06
  Bottom 0.203: U3.23 61.09,3.91 59.59,5.41 53.39,5.41 52.27,6.53 52.27,13.34 51.97,13.64 51.97,14.25 v52.78,15.06 53.7,15.98 53.7,25.22 50.44,28.47 50.44,33.05 49.83,33.66 49.83,39.24 48.82,40.26 | I2C.2 48.61,40.5 | 48.61,40.5 48.82,40.5 | 48.82,40.66 48.82,46.04 47.28,47.57 44.55,47.57 43.84,48.29 38.96,48.29 38.56,48.69 23.7,48.69 U3.17 | 48.82,40.66 48.82,40.5 | 48.61,40.5 48.78,40.66 48.82,40.66 | 48.82,40.26 48.82,40.5 | 48.61,40.5 48.61,40.46 48.82,40.26
BLE_SWCLK  (via drill 0.25 pad 0.51, 0.3 pad 0.51)
  Top 0.203: BLE1.26 v61.85,11.63 | U7.16 48.55,21.09 49.43,21.97 49.43,29.08 51.56,31.22 59.28,31.22 59.59,30.91 60.4,30.91 v60.71,31.22
  Bottom 0.203: v60.71,31.22 62.03,29.9 62.03,11.81 v61.85,11.63
BLE_SWDIO  (via drill 0.25 pad 0.51, 0.3 pad 0.51)
  Top 0.203: v60.58,11.63 BLE1.25 60.6,10.39 60.6,4.7 59.84,3.94 59.84,2.03 59.01,1.2 34.62,1.2 U3.30 | 47.86,21.87 U7.17 48.63,21.88 49.02,22.28 49.02,29.29 51.36,31.62 v59.99,31.62
  Bottom 0.203: v59.99,31.62 59.99,30.91 61.62,29.29 61.62,12.68 v60.58,11.63
BLE_TX  (via drill 0.25 pad 0.41, 0.25 pad 0.51)
  Top 0.203: BLE1.18 49.23,11.3 48.62,11.91 48.62,18.92 47.8,19.74 v47.4,19.74 | v43.03,34.37 43.84,35.18 57.25,35.18 57.56,35.48 57.56,38.95 UART.2 | U7.31 v44.05,27.04 v44.04,27.05
  Bottom 0.203: UART.2 54.81,41.69 54.81,43.51 55.63,44.32 55.63,48.59 56.24,49.2 58.78,49.2 59.59,50.01 60.17,50.01 U3.2 | v47.4,19.74 48.31,19.74 48.51,19.94 48.51,20.75 47.9,21.36 44.45,21.36 43.65,22.16 43.65,26.28 44.05,26.68 v44.05,27.04 | v44.05,27.04 44.05,33.56 44.75,34.27 44.75,34.67 44.25,35.18 43.84,35.18 v43.03,34.37 | v44.05,27.04 v44.04,27.05
BUTTON  (via drill 0.25 pad 0.51)
  Top 0.203: U7.3 41.83,24.38 v41.4,24.82 | RESET.2 21.97,4.06 | 22.4,4.5 22.4,4.24 22.1,3.94 | v38.25,8.15 37.64,8.15 34.19,4.7 31.65,4.7 30.89,3.94 22.1,3.94 | 22.2,3.58 RESET.2 | 22.1,3.94 RESET.2
  Bottom 0.203: v41.4,24.82 41.4,21.44 38.25,18.29 v38.25,8.15
CDC
  Top 0.203: U7.21 48.4,23.88 48.62,24.11 48.62,28.17 48.08,28.7 CDC.-
DAP  (via drill 0.25 pad 0.51)
  Top 0.203: U7.12 45.05,20.23 v44.86,20.04 | 44.98,28.7 DAP.- 44.42,27.86 43.74,27.86 43.33,27.46 42.6,27.46 v42.16,27.03
  Bottom 0.203: v42.16,27.03 42.16,26.47 42.8,25.83 42.8,21.49 44.25,20.04 v44.86,20.04
GND  (via drill 0.25 pad 0.51)
  Top 0.254: v27.89,39.95 27.87,39.98 U1.3 24.51,39.98 | U1.19 30.48,34.73 30.02,35.18 28.98,35.18 U1.16 | U1.29 33.31,37.48 33.27,37.52 | 27.48,41.08 U1.48 27.02,42.68 27.01,42.67
  Top 0.305: U1.9 27.25,36.98 27.28,37.01 | 27.99,35.28 27.98,35.27 U1.14 27.98,32.15 27.99,32.13
  Top 0.381: C16.1 C4.1
  Top 0.406: C18.1 35.2,13.84 37.03,15.67 v37.03,15.98
  Top 0.508: v61.32,7.54 62.2,7.54 62.26,7.49 | v61.32,6.63 62.15,6.63 62.26,6.73 | 13.26,43.41 13.49,43.64 J2.6 16.33,43.64 v16.41,43.71 | 40.49,27.05 40.47,27.04 C27.1 39.79,25.54 39.78,25.53 | 39.78,20.95 39.79,20.97 C28.1 40.47,20.36 40.49,20.34 | C4.1 35.56,29.72 C6.1 | v47.17,5.82 47.17,6.71 46.82,7.05 C20.- | C20.- 44.64,7.05 v44.55,6.96 | v46.33,5.84 46.33,7.02 C20.- | C20.- 46.36,7.92 v46.28,8
  Top 0.61: 63.12,10.01 BLE1.27 63.12,7.9 63.27,7.75 | v45.21,23.76 45.21,23.72 U7.33 | BLE1.1 63.12,20.8 62.76,20.45 60.6,20.45 60.48,20.32
  Top 0.635: C7.1 C8.1 R2.1 | C2.1 C3.1 19.96,40.51 | C2.1 R1.1 | R1.1 20.83,36.1 | 20.83,36.1 C1.1 20.83,34.42 C5.1 | C5.1 20.8,33.43 21.97,32.26 C17.2 | C5.1 17.96,34.39 17,33.44 14.74,33.44 | J2.G4 14.74,33.44 | 11.75,7.3 C26.1 | C13.1 20.89,27.95 v20.88,27.96 | C9.- 40.26,34.06 40.4,34.06 40.4,34.81 39.9,35.31 C10.1 | C2.1 19.96,38.99 | R1.1 19.96,37.47 | 20.83,36.1 20,36.1 19.96,36.07 | J2.G4 13.27,33.44 13.26,33.45 | 14.74,33.44 14.74,34.82 v14.68,34.87 | J2.G4 14.61,31.96 14.58,31.93 | C12.1 C11.1
  Top 0.762: 13.16,48.18 13.21,48.24 J2.G1 15.85,48.24 15.9,48.29 | C30.1 54.84,7.37 v54.81,7.34
  Bottom 0.508: 30.43,37.24 MODE0.2 | MODE0.2 30.38,37.21 | 30.38,37.21 29.62,37.21 v29.59,37.24 | MODE2.2 32.08,37.19 | 32.08,37.19 MODE1.2 MODE0.2 | MODE2.2 34.34,37.19 | MODE2.2 33.58,36.47 | 32.08,37.19 32.08,36.5 | v30.35,36.6 30.35,37.19 30.38,37.21
  Bottom 0.61: 30.53,11.2 30.53,10.69 29.08,9.25 POE_GND.2 29.08,9.75 30.53,11.2
  Bottom 0.635: v20.88,27.96 20.88,29.69 20.78,29.79
  other vias: 43.94,16.21 39.67,20.95 39.67,25.53 40.39,26.64 35.04,10.27 36.35,10.26 11.94,8.66 10.11,8.18 26.82,1.37 17.53,1.65 14.88,1.65 21.89,32.33 20.88,33.35 19.96,39.04 20.07,40.56 19.96,37.52 13.77,43.61 13.26,48.18 15.8,48.29 6.65,48.18 3.3,48.18 4.93,49.4 3.3,32.64 6.76,32.54 5.13,33.76 5.03,31.42 13.36,33.45 14.58,32.03 15.7,33.45 40.39,40.82 40.39,37.92 40.49,42.09 44.55,42.6 43.54,35.79 42.01,35.79 39.98,29.69 38.25,29.69 36.73,29.69 33.6,47.68 32.46,47.68 30.78,47.52 29.67,47.55 18.14,47.17 32.51,52.5 61.32,45.85 61.62,31.62 61.72,35.69 44.26,24.92 45.21,24.92 46.25,24.92 44.26,23.76 46.25,23.72 44.26,22.34 45.21,22.4 46.25,22.38 32.08,36.55 43.84,51.33 58.98,20.55 55.42,14.35 58.06,8.66 65.53,4.55 67.61,32.54 64.06,37.11 66.09,38.53 65.18,49.1 65.18,45.03 65.18,40.77 54.91,37.41 37.13,19.84 6.76,1.24 1.17,11.51 5.64,11.51 1.88,9.88 4.72,10.29 6.05,8.66 25.15,34.57 23.32,34.98 39.57,9.63 39.6,12.22 62.13,48.59 63.45,52.55 54.71,52.55 12.95,52.55 7.16,52.55 1.47,52.35 1.37,46.05 1.78,38.13 1.68,30.51 17.63,30.51 8.76,1.14 28.96,36.09 27.76,37.77 25.2,32.39 29.59,35.59 61.11,40.77 44.55,41.28 44.55,39.85 44.55,38.23 46.99,44.02 53.48,7.12 19.96,36.09 46.08,34.16 47.8,34.06 63.73,7.11 38.96,27.25 36.22,26.95 36.12,25.32 36.12,23.29 36.02,20.75 36.22,17.91 54.81,26.34 55.73,27.36 53.47,30.63 52.5,32.54 50.14,24.61 50.06,23.41 55.42,20.55 55.42,17.09 58.88,17.09 58.88,14.45 57.76,13.03 58.88,45.95 35.48,47.57 21.69,47.47 24.22,42.53 26.57,41.78 31.34,40.36 33.17,35.69 3,6.32 3,4.8 3,3.28 16.92,37.41 17.02,35.59 40.36,36.3 44.55,36.4 40.39,39.45 24.13,2.46 36.93,3.68 44.25,5.71 30.23,49.81 17.12,52.65 42.62,43.1 37.03,14.96 35.71,8.23 47.24,12.42 46.86,46.18 52.2,48.46 44.53,11.02 44.65,14.45 42.75,12.42
LINKLED  (via drill 0.25 pad 0.51)
  Top 0.203: U1.25 35.92,35.48 v36.32,35.08
  Bottom 0.203: v36.32,35.08 36.02,35.08 35.71,34.77 35.71,31.72 35.2,31.22 35.2,17.6 36.22,16.59 36.22,15.82 33.94,13.54 13.88,13.54 J1.9
MSD  (via drill 0.25 pad 0.51)
  Top 0.203: v41.5,26.44 41.5,27.36 42.01,27.86 42.9,27.86 MSD.- | U7.7 42.12,22.38 41.91,22.17 41.91,21.51 v42.68,20.74
  Bottom 0.203: v41.5,26.44 42.42,25.53 42.42,21.01 v42.68,20.74
N$1
  Top 0.254: R1.2 23.34,36.48 U1.10 23.49,36.48 22.5,37.47
N$2
  Top 0.203: J1.12 17.93,27.56 18.92,28.55 R16.1
N$4
  Top 0.203: J1.10 14.88,14.82 14.88,12.62 14.38,12.12 R17.1
N$5
  Top 0.203: R4.2 C12.2 42.24,41.4 X1.2
N$6
  Top 0.203: D1.+ R18.1
N$7
  cutout Top: 40.89,41.99 40.89,37.01 44.15,37.01 44.15,41.99
  cutout Top: 36.63,25.93 36.63,20.95 39.47,20.95 39.47,25.93
N$8  (via drill 0.3 pad 0.51)
  Top 0.508: R19.2 v23.37,14.35 | R20.2 v26.42,14.35
  Top 0.762: C13.2 22.33,18.29 23.37,17.25 R19.2 | R21.2 v29.59,16 | R22.1 v35.18,16.38
  Bottom 0.762: v23.37,14.35 v26.42,14.35 29.21,14.35 | 29.21,14.35 29.51,14.35 | 29.51,14.35 29.92,14.35 | 29.92,14.35 33.57,14.35 35.18,15.96 v35.18,16.38 | v29.59,16 29.59,14.73 | 29.59,14.68 29.59,14.43 29.51,14.35 | 29.59,14.73 29.21,14.35 | 29.59,14.73 29.59,14.68 | 29.59,14.68 29.92,14.35
N$9
  Top 0.254: C15.2 29.59,29.08 29.97,28.7 33.02,28.7 33.66,28.07 U2.1
N$10  (via drill 0.25 pad 0.51)
  Top 0.305: 18.17,12.31 U5.1 20.69,12.31 20.47,12.52 | 20.47,12.52 18.34,12.52 | 20.47,12.52 20.27,12.73 18.44,12.73
  Top 0.406: 18.34,12.52 17.25,12.52 v17.17,12.45
  Top 0.635: J1.4 14.74,20.19 J1.5
  Top 0.762: R30.2 18.44,12.73 18.44,13.74 17.93,14.25 17.93,14.71 C32.2 18.03,15.57 17.22,16.38 17.22,19.74 J1.5
  Bottom 0.406: v17.17,12.45 14.76,12.45 11.2,8.89 8.93,8.89 6.48,6.43 POE_IN.T
N$11
  Top 0.203: U2.10 26.04,16.26 R19.1
N$12
  Top 0.203: U7.14 46.05,19.95 R36.2
N$13
  Top 0.254: U2.3 31.12,27.56 30.73,27.94 28.32,27.94 C14.2
N$14
  Top 0.203: CDC.+ R42.1
N$15  (via drill 0.3 pad 0.51)
  Top 0.254: U2.2 v32.39,27.81 | C16.2 v31.88,29.72 R26.2 | v28.7,28.7 28.7,29.08 R27.2
  Bottom 0.254: v32.39,27.81 32.39,28.32 | 32.39,28.32 32.39,28.83 | 32.39,28.83 32.39,29.21 32.26,29.34 | 32.26,29.34 v31.88,29.72 | v28.7,28.7 32,28.7 | 32,28.7 32.26,28.7 32.39,28.83 | 32.39,28.32 32,28.7 | 32.26,29.34 32.26,28.96 32,28.7
N$16
  Top 0.203: U7.13 45.55,18.89 45.59,18.89 R37.2
N$17
  Top 0.203: U2.15 32.39,14.71 32.03,14.35 28.7,14.35 R20.1
N$18
  Top 0.305: R33.2 R34.1 20.19,10.39 20.61,10.81 U5.4
N$19
  Top 0.305: U5.2 19.86,11.81 19.08,11.02 R30.1 18.34,11.02 R31.2
N$20  (via drill 0.3 pad 0.51)
  Top 0.203: U2.7 v26.04,27.81 | R25.2 C17.1 v21.97,27.81
  Bottom 0.203: v26.04,27.81 v21.97,27.81
N$21  (via drill 0.25 pad 0.51)
  Top 0.203: J3.3 6.07,5.38 6.5,4.95 6.5,3.81 7.2,3.11 7.96,3.11 v8.41,2.67 8.42,2.65 D4.- | R36.1 v47.33,16.19 | R38.1 37.53,17.11 38.63,16 v39.52,16
  Bottom 0.203: v8.41,2.67 8.85,3.11 25.87,3.11 27.46,4.7 41.43,4.7 43.08,6.35 43.08,11.3 46.76,14.99 46.76,15.62 v47.33,16.19 46.51,17.02 40.54,17.02 v39.52,16
N$22  (via drill 0.25 pad 0.51)
  Top 0.203: R46.2 v51.77,30
  Bottom 0.203: U3.16 25.83,49.1 38.76,49.1 39.17,48.69 44.04,48.69 44.75,47.98 47.47,47.98 49.23,46.23 49.23,44.4 50.65,42.98 50.65,34.06 51.26,33.45 51.26,30.5 v51.77,30
N$23  (via drill 0.25 pad 0.51)
  Top 0.203: D6.- 9.12,3.94 v8.41,3.94 7.96,3.49 7.33,3.49 6.88,3.94 6.88,5.14 5.99,6.04 J3.2 | R37.1 v45.81,16.19
  Bottom 0.203: v8.41,3.94 8.85,3.49 25.74,3.49 27.33,5.08 41.3,5.08 42.7,6.48 42.7,11.43 46.38,15.11 46.38,15.62 v45.81,16.19
N$24
  Top 0.508: R28.1 PWR.+
N$25
  cutout Top: 0.25,29.08 35.31,29.08 35.31,14.55 0.25,14.55
  cutout Bottom: 0.25,29.08 35.61,29.18 35.61,14.66 0.25,14.66
N$26
  Top 0.203: 10,5.87 C25.2
  Top 0.305: J3.1 4.86,6.85 4.85,6.86 4.85,6.92
  Top 0.381: 11.75,5.78 C26.2
  Top 0.813: F1.1 13.91,5.78 11.75,5.78 C25.2 9.11,5.78 7.96,6.92 6.29,6.92 4.85,6.92 4.47,6.92
N$28
  Top 0.203: U7.4 40.61,23.88 C27.2 39.59,24.02 X2.2
N$29
  Top 0.203: X2.1 39.08,22.49 C28.2 41.37,23.38 U7.5
N$30
  Top 0.305: R32.2 23.65,6.22 24.28,6.86 24.28,10.29 23.27,11.31 U5.6
N$31
  Top 0.254: U7.9 43.55,20.13 44.25,19.43 44.25,18.69 R41.2 R40.2
N$32
  Top 0.305: R35.1 23.39,10.41 23,10.81 U5.5
N$33
  Top 0.203: MSD.+ R43.1
N$34
  Top 0.203: DAP.+ R44.1
N$35
  Top 0.203: L.+ R47.1
N$36
  Top 0.203: Q1.3 38.04,19.19 R38.2
N$37
  Top 0.152: 25.35,11.3 25.25,11.41
  Top 0.305: U5.8 24.65,12.31 | 24.65,12.31 25.96,12.31 | U5.8 24.35,12.31 25.13,11.53 | 25.13,11.53 25.25,11.41 | 24.65,12.31 25.15,11.81 | U5.8 23.52,13.03 | 23.52,13.03 25.65,13.03 | 23.52,12.73 23.42,12.73 23.42,12.52 | 23.52,12.73 25.55,12.73 | 23.11,12.52 23.42,12.52 | 23.42,12.52 25.25,12.52 | 23.52,13.03 23.52,12.73 | 25.13,11.53 25.13,12.24 25.04,12.32
  Top 0.508: 25.35,11.3 25.76,11.3 L1.1
N$38
  cutout Top: 63.55,22.78 68.73,22.78 68.73,9.98 63.45,9.98 63.45,13.94 63.45,22.78
  cutout Bottom: 63.55,22.78 68.73,22.78 68.73,9.98 63.45,9.98 63.45,13.94 63.45,22.78
N$39
  Top 0.813: R45.1 31.9,10.95 D2.-
P0.00
  Top 0.203: BLE1.10 50.55,22.78 51.77,24 R46.1
P0.01  (via drill 0.25 pad 0.51)
  Top 0.203: v52.48,20.24 50.6,20.24 BLE1.11
  Bottom 0.203: v52.48,20.24 51.77,19.53 51.77,18.41 50.24,16.89 50.24,12.83 50.65,12.42 50.65,2.95 U3.19
P0.02  (via drill 0.25 pad 0.51)
  Top 0.203: v52.48,18.92 BLE1.12
  Bottom 0.203: v52.48,18.92 52.48,18.41 50.65,16.59 50.65,13.03 51.05,12.62 51.05,5.08 U3.20
P0.03  (via drill 0.25 pad 0.51)
  Top 0.203: v52.58,17.6 50.6,17.6 BLE1.13
  Bottom 0.203: U3.21 56.01,4.01 55.42,4.6 52.98,4.6 51.46,6.12 51.46,12.83 51.05,13.23 51.05,16.08 v52.58,17.6
P0.04  (via drill 0.25 pad 0.51)
  Top 0.203: v52.68,16.38 BLE1.14
  Bottom 0.203: U3.22 58.55,3.91 57.45,5 53.19,5 51.87,6.33 51.87,13.03 51.46,13.44 51.46,15.16 v52.68,16.38
P0.10  (via drill 0.3 pad 0.51)
  Top 0.203: BLE1.20 54.23,11.63 56.03,13.44 v56.77,13.44
  Bottom 0.203: U3.4 54.31,49.23 54.31,35.87 61.21,28.96 61.21,13.54 59.79,12.12 59.79,10.9 58.98,10.08 56.44,10.08 55.63,10.9 55.63,12.83 56.24,13.44 v56.77,13.44
P0.12  (via drill 0.3 pad 0.51)
  Top 0.203: BLE1.22 v56.77,11.61
  Bottom 0.203: U3.6 53.49,48.36 53.49,35.48 60.4,28.57 60.4,13.95 58.98,12.52 58.98,11.3 58.57,10.9 57.48,10.9 v56.77,11.61
P0.13  (via drill 0.3 pad 0.51)
  Top 0.203: BLE1.23 v58.04,11.61
  Bottom 0.203: U3.7 53.09,46.23 53.09,35.28 59.94,28.42 59.94,14.1 58.04,12.19 v58.04,11.61
P0.18  (via drill 0.3 pad 0.51)
  Top 0.203: BLE1.2 61.85,22.88 | 61.85,22.88 61.85,23.37 | v59.18,25.65 60.27,25.65 61.82,24.11 61.82,22.91 61.85,22.88
  Bottom 0.203: U3.9 42.8,49.91 44.86,49.91 45.57,49.2 48.11,49.2 52.27,45.04 52.27,34.87 57.45,29.69 57.45,25.12 57.76,24.82 58.88,24.82 59.18,25.12 v59.18,25.65
P0.23  (via drill 0.3 pad 0.51)
  Top 0.203: BLE1.4 59.31,23.68 v59.32,23.7
  Bottom 0.203: U3.10 40.67,49.51 44.6,49.51 45.31,48.79 47.89,48.79 51.87,44.81 51.87,34.67 57.05,29.49 57.05,24.82 57.56,24.31 58.71,24.31 v59.32,23.7
P0.30  (via drill 0.25 pad 0.51)
  Top 0.152: 52.93,22.38 BLE1.9
  Top 0.203: 52.93,22.38 52.93,23.65 v52.98,23.7 53.3,24.02 R47.2
  Bottom 0.203: v52.98,23.7 52.98,21.77 51.36,20.14 51.36,18.62 49.83,17.09 49.83,12.62 50.24,12.22 50.24,3.86 47.78,1.4 29.34,1.4 U3.32
PD2/INT  (via drill 0.25 pad 0.51, 0.3 pad 0.51)
  Top 0.203: U1.36 35.2,40.97 35.51,41.28 35.51,42.02 38.44,44.96 R6.2 39.48,44.96 v39.54,44.91 | v55.02,45.54 54.95,45.48 v49.78,45.48 43.59,45.48 v42.76,46.3 | BLE1.19 52.96,10.77 52.98,10.79 52.98,12.73 v53.49,13.23
  Bottom 0.203: v55.02,45.54 55.02,48.79 55.83,49.61 57.23,49.61 U3.3 | v53.49,13.23 54.51,14.25 54.51,25.63 52.48,27.66 52.48,30.4 51.66,31.22 51.66,33.66 51.05,34.27 51.05,43.33 49.78,44.6 v49.78,45.48 | v39.54,44.91 39.54,45.4 40.44,46.3 v42.76,46.3
PMODE0  (via drill 0.25 pad 0.51, 0.3 pad 0.51)
  Top 0.203: U1.45 28.98,41.22 v28.65,40.89 | v26.37,42.8 25.96,43.21 23.52,43.21 R13.2
  Bottom 0.203: MODE0.1 30.4,38.56 28.65,40.31 v28.65,40.89 28.65,42.44 27.89,43.21 26.77,43.21 v26.37,42.8
PMODE1  (via drill 0.3 pad 0.51)
  Top 0.203: v29.51,40.89 29.48,40.93 U1.44 29.48,43.55 29.21,43.82 23.52,43.82 23.27,43.56 R14.2
  Bottom 0.203: MODE1.1 31.9,37.97 29.51,40.36 v29.51,40.89
PMODE2  (via drill 0.3 pad 0.51)
  Top 0.203: R15.2 23.27,45.19 24.23,44.22 29.52,44.22 29.98,43.77 U1.43 29.98,41.58 30.4,41.15 v30.4,40.7
  Bottom 0.203: MODE2.1 33.58,38.33 33.05,38.86 31.77,38.86 30.4,40.23 v30.4,40.7
POE_OUT  (via drill 0.25 pad 0.51)
  Top 0.508: R33.1 v22.48,7.75 | 28.83,7.75 28.83,7.64 28.98,7.49 | 29.16,9.32 29.16,11.1 L1.2
  Top 1.016: 29.16,9.32 28.83,8.99 28.83,7.75 | C31.+ 28.88,7.49 28.98,7.49 v30.61,7.49 D2.+ 31.75,8.1 33.68,10.03 D7.-
  Bottom 0.508: v22.48,7.75 24.28,7.75 24.92,8.38 26.19,8.38 27.08,7.49 v30.61,7.49
PROG_RESET  (via drill 0.25 pad 0.51)
  Top 0.203: C29.2 R39.1 44.77,15.62 42.44,15.62 41.81,16.26 41.81,19.53 42.21,19.94 v42.72,19.94 | U7.2 42.25,24.88 v41.5,25.63
  Bottom 0.203: v41.5,25.63 41.71,25.63 42.01,25.32 42.01,20.23 42.3,19.94 v42.72,19.94 42.72,19.43 43.23,18.92 PROG_RESET.T
RX1_N  (via drill 0.3 pad 0.51)
  Top 0.203: R26.1 v30.35,31.24 C15.1
  Top 0.254: v27.05,39.17 27.05,38.99 25.79,38.99 U1.5
  Bottom 0.254: v27.05,39.17 27.05,38.99 27.98,38.99 arc-90 28.96,38.02 28.96,37.59 arc-90 27.94,36.58 26.8,36.58 arc90 26.44,36.22 26.44,36.02 arc90 26.9,35.56 27.73,35.56 arc-90 28.47,34.82 28.47,34.38 arc-90 27.62,33.53 26.8,33.53 arc90 26.44,33.17 26.44,32.84 arc90 26.9,32.39 29.2,32.39 arc-90 29.72,31.86 29.72,31.44 29.92,31.24 v30.35,31.24
RX1_P  (via drill 0.3 pad 0.51)
  Top 0.203: C14.1 v27.31,31.24 R27.1
  Top 0.254: v27.05,38.3 27.05,38.48 U1.6
  Bottom 0.254: v27.05,38.3 27.05,38.48 28.01,38.48 arc-90 28.45,38.04 28.45,37.64 arc-90 27.89,37.08 26.75,37.08 arc90 25.93,36.27 25.93,35.97 arc90 26.85,35.05 27.61,35.05 arc-90 27.97,34.69 27.97,34.4 arc-90 27.61,34.04 26.74,34.04 arc90 25.93,33.23 25.93,32.78 arc90 26.83,31.88 28.87,31.88 arc-90 29.21,31.54 29.21,31.4 29.05,31.24 v27.31,31.24
RX_N  (via drill 0.3 pad 0.51)
  Top 0.254: U2.16 v33.66,16.38 R22.2
  Bottom 0.254: J1.6 16.07,22.23 arc-45 16.83,21.92 17.18,21.56 arc45 18.04,21.21 21.53,21.21 arc-45 22.72,20.71 24.08,19.35 arc45 24.82,19.05 31.98,19.05 arc-90 33.43,17.6 33.43,16.61 v33.66,16.38
RX_P  (via drill 0.3 pad 0.51)
  Top 0.254: U2.14 v31.12,16.38 R21.1
  Bottom 0.254: J1.3 16.9,20.31 arc-45 17.83,20.7 21.33,20.7 arc-45 22.51,20.21 23.86,18.86 arc45 24.62,18.54 31.93,18.54 arc-90 32.92,17.55 32.92,17.09 arc-90 32.21,16.38 v31.12,16.38
SD_SS  (via drill 0.25 pad 0.51, 0.3 pad 0.51)
  Top 0.203: J2.2 16.26,39.24 17.4,38.1 17.78,37.72 R29.2 18.54,36.8 18.24,36.5 v15.39,36.5 | U3.5 51.94,52.45 33.78,52.45 32.97,51.64 32.97,49.91 31.14,48.08 v19.96,48.08 | BLE1.21 55.5,11.99 56.03,12.52 v56.82,12.52
  Bottom 0.203: U3.5 53.9,50.5 53.9,35.69 60.81,28.78 60.81,13.74 59.39,12.32 59.39,11.1 58.78,10.49 56.64,10.49 56.03,11.1 56.03,12.32 56.24,12.52 v56.82,12.52 | v19.96,48.08 16.81,48.08 15.39,46.66 v15.39,36.5
SPDLED  (via drill 0.25 pad 0.51)
  Top 0.203: U1.24 33.7,33.78 v34.19,34.27 | v34.19,28.47 41.99,28.47 D1.-
  Bottom 0.203: v34.19,34.27 34.9,33.55 34.9,32.13 34.19,31.42 v34.19,28.47
TOCAP  (via drill 0.25 pad 0.51, 0.3 pad 0.51)
  Top 0.203: C7.2 37.64,31.27 37.03,31.88 36.22,31.88 35.56,32.54 v34.19,32.54 | U1.20 30.98,35.14 v30.53,35.59
  Bottom 0.203: v34.19,32.54 32.95,32.54 arc-90 30.53,34.96 v30.53,35.59
TX1_N  (via drill 0.3 pad 0.51)
  Top 0.203: R24.2 24.68,29.37
  Top 0.254: U1.1 24.67,40.98 24.51,41.14 24.51,41.56 v24.67,41.72 | U2.6 27.31,27.84 26.57,28.57 24.74,28.57 v24.68,28.51 24.68,29.37
  Bottom 0.203: 24.51,41.58 24.53,41.58 | 24.51,28.57 24.61,28.57
  Bottom 0.254: 24.51,28.57 24.51,41.58 | 24.53,41.58 v24.67,41.72 | 24.61,28.57 v24.68,28.51
TX1_P  (via drill 0.3 pad 0.51)
  Top 0.203: U2.8 24.77,27.05 | R23.2 23.84,29.37
  Top 0.254: U1.2 24.5,40.48 24,40.98 24,41.56 v23.84,41.72 | 24.77,27.05 23.84,27.98 v23.84,28.51 23.84,29.72 R23.2
  Bottom 0.203: 24,41.58 23.98,41.58 | 24,28.57 23.91,28.57
  Bottom 0.254: 24,28.57 24,41.58 | 23.98,41.58 v23.84,41.72 | 23.91,28.57 v23.84,28.51
TX_N  (via drill 0.3 pad 0.51)
  Top 0.254: v27.31,16.7 U2.11
  Bottom 0.152: 14.7,18.16 14.67,18.16 arc90 J1.2
  Bottom 0.254: 14.7,18.16 16.81,18.16 arc-90 17.81,17.17 17.81,15.44 arc90 18.26,14.99 18.79,14.99 arc90 19.33,15.53 19.33,18.44 arc-90 20.32,19.43 20.88,19.43 arc-90 21.87,18.44 21.87,16.46 arc90 22.33,16 23.01,16 arc90 23.39,16.38 23.39,16.63 arc-90 24.42,17.65 25.87,17.65 arc-90 26.44,17.08 arc90 26.83,16.7 v27.31,16.7
TX_P  (via drill 0.3 pad 0.51)
  Top 0.254: U2.9 v24.77,16.26
  Bottom 0.254: J1.1 15.76,17.65 16.76,17.65 arc-90 17.3,17.11 17.3,15.33 arc90 18.15,14.48 18.87,14.48 arc90 19.84,15.45 19.84,18.36 arc-90 20.41,18.92 20.82,18.92 arc-90 21.36,18.38 21.36,16.35 arc90 22.21,15.49 23.22,15.49 arc90 23.9,16.18 23.9,16.61 arc-90 24.44,17.14 25.53,17.14 arc-90 25.93,16.74 25.93,16.61 arc-90 25.57,16.26 v24.77,16.26
USB_CONNECT  (via drill 0.25 pad 0.51)
  Top 0.203: v39.07,18.11 39.07,17.17 Q1.1 | v46.69,20.14 46.55,20.28 U7.15
  Bottom 0.203: 39.27,17.91 v39.07,18.11 39.52,17.65 45.92,17.65 46.69,18.41 v46.69,20.14
VCC
  Top 0.305: U5.3 20.22,11.31 19.01,10.1 18.95,10.03 18.59,9.68 18.59,9.5 | C23.2 18.59,9.5 | 18.59,9.5 19.27,8.83 19.27,7.15 R32.1
VCC1
  Top 0.508: D5.- 64.29,33.66 66.17,31.77 U3.39
W_REST  (via drill 0.25 pad 0.51, 0.3 pad 0.51)
  Top 0.203: BLE1.3 60.58,23.42 59.39,24.61 58.37,24.61 58.17,24.82 v58.17,25.53 | U1.37 34.68,42.68 35.7,43.7 v35.95,43.96 R7.2 | v49.94,48.41 42.72,48.41 40.79,46.48 v40.79,45.59
  Bottom 0.203: v58.17,25.53 58.17,29.59 52.68,35.08 52.68,45.67 v49.94,48.41 48.74,49.61 47.17,49.61 U3.8 | v40.79,45.59 40.79,44.96 39.78,43.94 35.97,43.94 v35.95,43.96
WSS  (via drill 0.25 pad 0.51, 0.3 pad 0.51)
  Top 0.203: U1.32 36.18,38.98 36.83,39.62 36.83,41.76 37.74,42.67 39.55,42.67 40.89,44.02 R5.2 42.67,44.93 48.92,44.93 49.23,44.63 v50.95,44.63 | BLE1.5 58.04,23.37 v58.29,23.62
  Bottom 0.203: U3.11 38.1,49.53 39.04,49.53 39.47,49.1 44.35,49.1 45.06,48.39 47.66,48.39 50.95,45.09 v50.95,44.63 51.46,44.12 51.46,34.47 56.64,29.29 56.64,24.11 57.12,23.62 v58.29,23.62
XI
  Top 0.203: U1.30 36.57,37.98 R3.2 C11.2 42.04,36.83 42.42,37.21 | 42.8,37.21 42.42,37.21 | 42.42,37.21 42.42,37.26 X1.1
  Top 0.254: 42.37,37.21 X1.1
XO
  Top 0.203: U1.31 36.57,38.48 36.7,38.35 R3.1 R4.1
(copper drawn outside any net)
  shapes: Bottom circle x1

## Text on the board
Bottom: B
tPlace: P6 | P5 | P0 | P9 | P8 | P7 | GND | P29 | P28 | P25 | P24 | P23 | P18 | P17 | P13 | P12 | P11 | P10 | SCL | RX | SDA | TX | 3V3 | 3V3 | GND | GND | L | MISO | VCC | MSD | DAP | CDC | D1 | SCK | MOSI | NC | GND | ANALOG | P30 | 3V3 | !RST | 3V3 | 5V | GND | GND | NC | P1 | P2 | P3 | P4 | P5 | P6 | PWR
bPlace: P6 | P5 | P0 | P9 | P8 | P7 | GND | P29 | P28 | P25 | P24 | P23 | P18 | P17 | P13 | P12 | P11 | P10 | P6 | P7 | P5 | P8 | 3V3 | 3V3 | GND | GND | V1.0 | 05/28/2015 | P30 | 3V3 | !RST | 3V3 | 5V | GND | GND | VIN | P1 | P2 | P3 | P4 | P5 | P6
